ORGANIZATION_BLOCK MAIN:OB1
TITLE= Miscelatore di due liquidi
// Simulatore: 12
// Versione: 1.0
// Data: 24/01/2002
// Il processo di miscelazione e scarico del prodotto avviene
// completamente in automatico.
// Il ciclo viene avviato agendo sul pulsante di start (SB11)
// e può essere interrotto in qualsiasi momento dal pulsante
// di Stop (SB10). Dopo un arresto, al successivo riavvio,
// il ciclo riprenderà dalla fase in cui era stato interrotto,
// e la fase stessa verrà completata prima di passare alla
// successiva.
// Due contatori software (C1 e C2) provvedono a contare gli
// impulsi forniti dai traduttori di flusso (TF1, TF2) e
// quindi a contare i litri di prodotto che transitano nelle
// rispettive tubazioni verso il serbatoio.
// Ogni contatore sarà preimpostato sui litri di prodotto da
// caricare nel serbatoio (C1=60, C2=100) tenendo presente che
// la capacità massima (virtuale) del sebatoio è di 160 litri.
// Le fasi del processo sono così suddivise:
// 1) Carico della quantità impostata dei due prodotti
//    operata dall'apertura delle elettrovalvole  (YV1, YV2)
//    e dalla messa in funzione delle pompe (P1, P2)
// 2) Quando il carico è completato inizia una fase di
//    riscaldamento (apertura dell'elettrovalvola YV4 che
//    immette vapore nel serbatoio) e mescolazione (motore M3
//    che aziona un mescolatore). La durata di questa fase è
//    gestita dal temporizzatore T32.
// 3) Trascorso il tempo della fase precedente viene
//    avviato lo scarico del prodotto (elettrovalvola YV3)
//    e quando il serbatoio si è completamente svuotato
//    riprende un nuovo ciclo.
// Le informazione sul livello (Minimo, Massimo) del serbatoio
// vengono ricavate dai due bit (TL1,TL2) del trasduttore
// di livello e vengono memorizzate in due marker
// M1.0 (Minimo) e M1.1 (Massimo), il marker M0.1 memorizzerà
// la condizione di carico dei prodotti completata (che può
// non corrispondere alla condizione di serbatoio pieno).
// Quattro lampade segnalono rispettivamente:
//   HL1: Pompa P1 in funzione
//   HL2: Pompa P2 in funzione
//   HL3: Fase di riscaldamento e miscelazione
//   HL4: Fase di scarico
//

BEGIN
NETWORK 1 //Resetta Marker alto livello al primo ciclo
//
LD SM0.1
R M0.2 1
R M0.1 1

NETWORK 2 //Imposta Merker  Serbatoio Pieno
//
LD I0.2
A I0.3
= M1.1

NETWORK 3 //Imposta Merker Serbatoio Vuoto
//
LDN I0.2
AN I0.3
= M1.0

NETWORK 4 //Conteggio Litri Prodotto 1
//
LD I0.0
LD M1.0
CTU C1 +60

NETWORK 5 //Conteggio Litri Prodotto 2
//
LD I0.1
LD M1.0
CTU C2 +100

NETWORK 6 //Imposta marker ON automatico
//
LD I0.6
O M0.2
A I0.7
= M0.2

NETWORK 7 //Riempimento prodotto 1
//
LD M0.2
AN C1
AN M1.1
= Q0.1
= Q0.0

NETWORK 8 //Riempimento prodotto 2
//
LD M0.2
AN C2
AN M1.1
= Q0.2
= Q0.3

NETWORK 9 //Imposta memoria serbatoio pieno
//
LD C1
A C2
O M1.1
EU
S M0.1 1

NETWORK 10 //Avvia Temporizzatore Miscelazione
//
LD M0.2
A M0.1
TON T32 +200

NETWORK 11 //Mescolazione e riscaldamento
//
LD M0.2
AN Q0.4
A M0.1
= Q0.5
= Q1.6

NETWORK 12 //Attiva fase di scarico
//
LD T32
EU
S M2.0 1
R M0.1 1

NETWORK 13 //Scarico miscela
//
LD M2.0
O Q0.4
A M0.2
AN M1.0
= Q0.4

NETWORK 14 //Reset Marker fase scarico
//
LD M1.0
EU
R M2.0 1

NETWORK 15 //Segalazione Pompa P1 in funzione
//
LD Q0.1
= Q0.6

NETWORK 16 //Segnalazione Pompa P2 in funzione
//
LD Q0.2
= Q0.7

NETWORK 17 //Segalazione Motore Mescolatore in Funzione
//
LD Q0.5
= Q1.0

NETWORK 18 //Segnalazione Scarico
//
LD Q0.4
= Q1.1

END_ORGANIZATION_BLOCK

